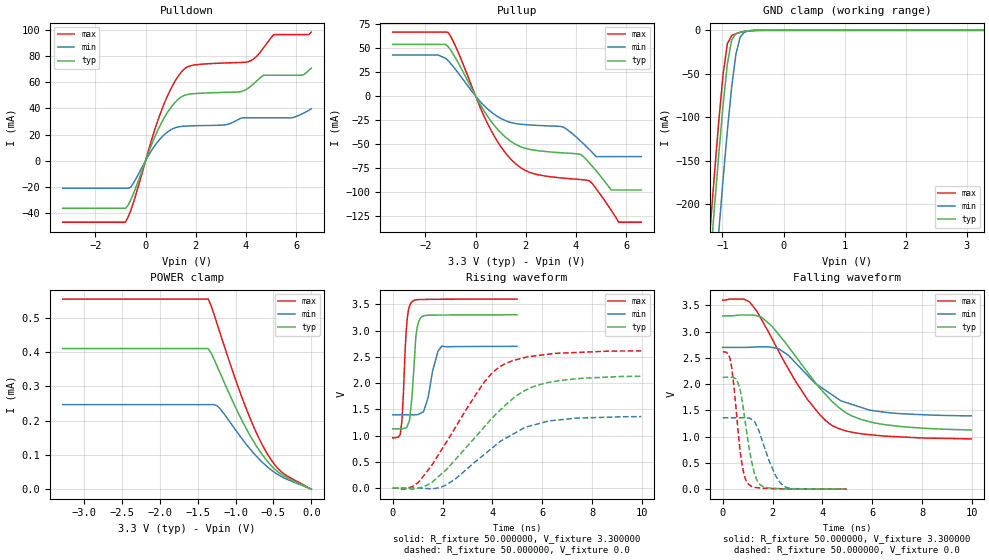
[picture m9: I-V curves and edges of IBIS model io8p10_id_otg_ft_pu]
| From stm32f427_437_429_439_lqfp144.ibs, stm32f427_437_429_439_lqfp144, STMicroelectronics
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|   Model io8p10_id_otg_ft_pu
[Model]  io8p10_id_otg_ft_pu
Model_type I/O
Polarity   Non-Inverting
Enable   Active-Low
Vinl =   0.990000V
Vinh =   2.310000V
Vmeas =  1.650000V
Cref =   40.000000pF
Rref =   100.000000M
Vref =   0.0V
C_comp   2.283100pF   2.214500pF   2.357400pF
[Temperature Range]   25.000000   0.125000k   -40.000000
[Pullup Reference]   3.300000V   2.700000V   3.600000V
[Pulldown Reference]   0.0V   0.0V   0.0V
[POWER Clamp Reference]   3.300000V   2.700000V   3.600000V
[GND Clamp Reference]   0.0V   0.0V   0.0V
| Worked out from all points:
|   slope of the pulldown table from 0 to 0.495 V, typ, clamps not added: 20.9 ohm
|   slope of the pullup table from 0 to 0.495 V, typ, clamps not added: 22.6 ohm
|   GND clamp passes 1 mA (typ) near -0.62 V on its own axis
|   rising waveform, R_fixture 50.000000, V_fixture 3.300000: 20-80 % time 193ps typ, 345ps min, 163ps max; typ from 1.13 V to 3.3 V
|   rising waveform, R_fixture 50.000000, V_fixture 0.0: 20-80 % time 2.52ns typ, 2.3ns min, 2.11ns max; typ from 0.005 V to 2.13 V
|   falling waveform, R_fixture 50.000000, V_fixture 3.300000: 20-80 % time 2.26ns typ, 2.05ns min, 2.03ns max; typ from 3.3 V to 1.13 V
|   falling waveform, R_fixture 50.000000, V_fixture 0.0: 20-80 % time 436ps typ, 637ps min, 341ps max; typ from 2.13 V to 0.005 V
[Pulldown]
|Voltage   I(typ)   I(min)   I(max)
-3.3V     -36.46mA   -21.09mA   -47.09mA
-800mV    -36.46mA   -21.09mA   -47.09mA
-600mV    -30.5mA    -20.54mA   -38.69mA
700mV     31.4mA     19.11mA    41.71mA
1.2V      45.15mA    25.37mA    61.75mA
1.6V      50.35mA    26.5mA     71.05mA
3.1V      52.28mA    27.26mA    74.75mA
4.1V      55.64mA    32.83mA    75.8mA
4.7V      65.4mA     32.83mA    86.49mA
5.1V      65.4mA     32.83mA    96.56mA
6.2V      65.4mA     35.57mA    96.56mA
6.6V      70.92mA    39.71mA    98.46mA
[Pullup]
|Voltage   I(typ)   I(min)   I(max)
-3.3V     54.05mA    42.89mA    66.92mA
-1.1V     51.84mA    37.2mA     66.69mA
500mV     -22.06mA   -13.99mA   -30.02mA
1.5V      -49.09mA   -28.3mA    -68.55mA
2.2V      -56.03mA   -30.32mA   -80.33mA
3.5V      -59.51mA   -32.64mA   -85.89mA
4.2V      -61.41mA   -47.48mA   -87.43mA
4.5V      -69.05mA   -55.11mA   -88.35mA
4.8V      -78.2mA    -63.4mA    -96.8mA
5.4V      -98.3mA    -63.4mA    -119.5mA
5.7V      -98.3mA    -63.4mA    -132mA
6.6V      -98.3mA    -63.4mA    -132mA
[GND_clamp]
|Voltage   I(typ)   I(min)   I(max)
-3.3V     -2.318A    -2.397A    -2.291A
-1.2V     -265.5mA   -356.1mA   -227.2mA
-1.13V    -202.7mA   -292.9mA   -164.1mA
-1.06V    -142.2mA   -231.2mA   -104.1mA
-990mV    -85.98mA   -171.6mA   -50.73mA
-920mV    -38.81mA   -115.5mA   -15.3mA
-850mV    -11.1mA    -65.61mA   -6.021mA
-780mV    -3.796mA   -27.43mA   -3.892mA
-710mV    -2.096mA   -7.699mA   -2.393mA
-640mV    -1.154mA   -2.125mA   -1.227mA
-570mV    -528.1uA   -803.6uA   -480.7uA
3.28V     0A         0A         0A
[POWER_clamp]
|Voltage   I(typ)   I(min)   I(max)
-3.28V    410.1uA    246.5uA    554.5uA
-1.36V    410.1uA    246.5uA    554.5uA
-1.32V    396.3uA    246.5uA    534.1uA
-1.28V    377.3uA    246.5uA    507.5uA
-1.2V     337.1uA    233.5uA    452.5uA
-1.04V    257.7uA    185.3uA    345.3uA
-880mV    185.4uA    137uA      247uA
-760mV    138.3uA    104.8uA    181.8uA
-640mV    98.44uA    77.14uA    126.4uA
-520mV    66.65uA    54.47uA    82.45uA
-400mV    43.68uA    37.32uA    51.43uA
0V        0A         0A         0A
[Ramp]
| variable   typ   min   max
dV/dt_r  1.26642/2.52306n   0.81168/2.30040n   1.56297/2.11421n
dV/dt_f  1.27992/2.24440n   0.77328/2.03555n   1.57182/2.03424n
R_load = 50.000000
[Rising Waveform]
R_fixture= 50.000000
V_fixture= 3.300000
V_fixture_min= 2.700000
V_fixture_max= 3.600000
|time   V(typ)   V(min)   V(max)
0s        1.129V     1.397V     959.6mV
300.3ps   1.131V     1.397V     1.022V
370.4ps   1.133V     1.397V     1.288V
500.5ps   1.147V     1.397V     2.651V
580.6ps   1.176V     1.397V     3.213V
760.8ps   1.682V     1.396V     3.542V
940.9ps   2.93V      1.399V     3.585V
1.171ns   3.263V     1.44V      3.591V
1.972ns   3.296V     2.707V     3.596V
4.985ns   3.3V       2.7V       3.599V
[Rising Waveform]
R_fixture= 50.000000
V_fixture= 0.0
V_fixture_min= 0.0
V_fixture_max= 0.0
|time   V(typ)   V(min)   V(max)
0s        4.838mV    4.389mV    5.42mV
780.8ps   -15.79mV   4.174mV    30.29mV
1.041ns   4.973mV    2.333mV    118mV
1.542ns   98.41mV    -10.77mV   417.7mV
2.162ns   360.2mV    67.41mV    885.3mV
3.624ns   1.14V      624.9mV    1.986V
4.404ns   1.53V      917.9mV    2.342V
5.245ns   1.845V     1.142V     2.481V
6.126ns   2V         1.263V     2.543V
9.97ns    2.131V     1.363V     2.614V
[Falling Waveform]
R_fixture= 50.000000
V_fixture= 3.300000
V_fixture_min= 2.700000
V_fixture_max= 3.600000
|time   V(typ)   V(min)   V(max)
0s        3.3V       2.7V       3.599V
880.9ps   3.315V     2.7V       3.612V
1.081ns   3.315V     2.702V     3.562V
1.542ns   3.278V     2.711V     3.243V
2.242ns   2.948V     2.674V     2.628V
3.403ns   2.225V     2.167V     1.708V
4.424ns   1.655V     1.785V     1.206V
5.185ns   1.395V     1.615V     1.087V
6.026ns   1.271V     1.498V     1.034V
9.97ns    1.129V     1.397V     959.6mV
[Falling Waveform]
R_fixture= 50.000000
V_fixture= 0.0
V_fixture_min= 0.0
V_fixture_max= 0.0
|time   V(typ)   V(min)   V(max)
0s        2.131V     1.363V     2.614V
300.3ps   2.132V     1.362V     2.476V
620.6ps   2.018V     1.362V     1.09V
840.8ps   1.493V     1.364V     310.2mV
1.031ns   867.5mV    1.357V     101.8mV
1.261ns   323.5mV    1.292V     40.93mV
1.451ns   114.9mV    1.118V     29.53mV
1.882ns   26.54mV    517.3mV    17.7mV
2.432ns   12.59mV    70.58mV    11.25mV
4.985ns   4.838mV    4.389mV    5.42mV
